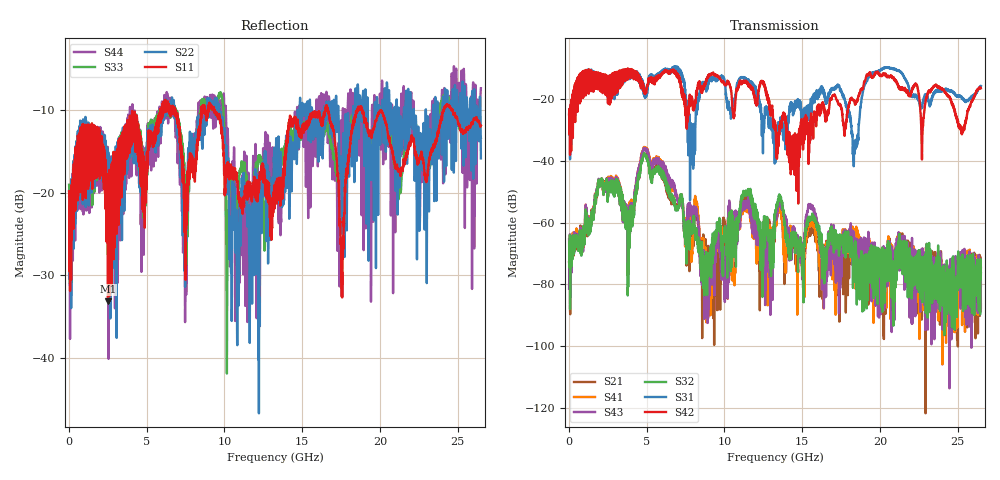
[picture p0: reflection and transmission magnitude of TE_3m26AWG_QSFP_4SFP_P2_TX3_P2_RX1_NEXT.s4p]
!Agilent Technologies,N5222A,MY51421691,A.10.00.00
!Agilent N5222A: A.10.00.00
!Date: Friday, January 30, 2015 12:35:16
!Correction: S11(Full 4 Port(1,2,3,4))
!S12(Full 4 Port(1,2,3,4))
!S13(Full 4 Port(1,2,3,4))
!S14(Full 4 Port(1,2,3,4))
!S21(Full 4 Port(1,2,3,4))
!S22(Full 4 Port(1,2,3,4))
!S23(Full 4 Port(1,2,3,4))
!S24(Full 4 Port(1,2,3,4))
!S31(Full 4 Port(1,2,3,4))
!S32(Full 4 Port(1,2,3,4))
!S33(Full 4 Port(1,2,3,4))
!S34(Full 4 Port(1,2,3,4))
!S41(Full 4 Port(1,2,3,4))
!S42(Full 4 Port(1,2,3,4))
!S43(Full 4 Port(1,2,3,4))
!S44(Full 4 Port(1,2,3,4))
!S4P File: Measurements: <S11,S12,S13,S14>,
!<S21,S22,S23,S24>,
!<S31,S32,S33,S34>,
!<S41,S42,S43,S44>:
# Hz S  dB  R 50.0
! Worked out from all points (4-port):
!   2650 points, 10 MHz to 26.5 GHz, reference 50 ohm
!   strongest paths, dB at 10 MHz, 6.63 GHz, 13.26 GHz, 19.88 GHz, 26.5 GHz:
!     S42: -24.8, -11.3, -27.5, -11.4, -16.4
!     S31: -24.9, -10.4, -34.2, -10.8, -15.7
!     S32: -72.9, -52.9, -56.9, -76.3, -76.4
!     S43: -81.4, -47.8, -58.8, -90.4, -80.4
!     S41: -72.9, -48.5, -61.5, -81.7, -87.5
!     S21: -65.4, -53.8, -61.0, -73.1, -74.7
!   lowest |S11| = -33.2 dB at 2.51 GHz (marker M1), VSWR 1.04, Z = 51 - j1.97 ohm
!   |S11| at or under -10 dB: start of sweep to 5.869 GHz; 9.355 GHz to 16.5 GHz (7.144 GHz wide, 55.3 % of centre); 18.85 GHz to 24.1 GHz (5.249 GHz wide, 24.4 % of centre)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
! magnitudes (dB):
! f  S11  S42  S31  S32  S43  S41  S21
! 10 MHz  -19.8  -24.8  -24.9  -72.9  -81.4  -72.9  -65.4
! 2.51 GHz  -33.2  -21.4  -19.7  -50.9  -47.7  -47.2  -50.2
! 5.8 GHz  -10.5  -12.7  -12.0  -43.3  -40.7  -40.3  -42.9
! 8.94 GHz  -10.3  -12.5  -15.8  -69.9  -82.1  -78.2  -69.5
! 11.46 GHz  -19.6  -14.5  -14.5  -50.2  -55.3  -56.4  -51.6
! 14.32 GHz  -11.9  -42.3  -21.0  -63.2  -66.4  -62.3  -64.7
! 26.5 GHz  -11.9  -16.4  -15.7  -76.4  -80.4  -87.5  -74.7
